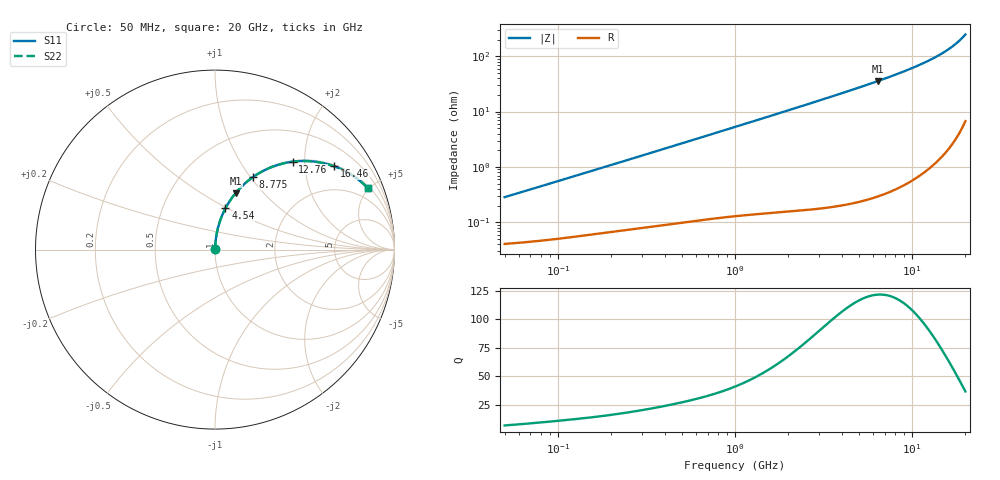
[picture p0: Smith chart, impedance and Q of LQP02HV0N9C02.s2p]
!Murata Part Number: LQP02HV0N9C02
!These Parameters are Measured in Series Mode Connection
!  o--[Z]--o
!Port1  Port2
!  o-------o
!Freq. Start=50[MHz] Stop=20[GHz], 401[Steps]
# Hz S RI R 50
!Freq.(Hz) S11(Real) S11(Imag) S21(Real) S21(Imag) S12(Real) S12(Imag) S22(Real) S22(Imag)
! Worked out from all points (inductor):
!   401 points, 50 MHz to 20 GHz, reference 50 ohm
!   read as one part in series: L = 889 pH near 51.52 MHz
!   highest Q = 121 at 6.407 GHz (marker M1), where L = 884 pH
!   S11 on the Smith chart (normalised r, x): 50 MHz: 1.00, +0.01; 4.54 GHz: 1.00, +0.49; 8.775 GHz: 1.01, +1.03; 12.76 GHz: 1.02, +1.74; 16.46 GHz: 1.05, +2.82; 20 GHz: 1.13, +4.94
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5e7  0.000415 0.00281  0.9996 -0.00281  0.9996 -0.00281  0.000415 0.00281
1.364002e8  0.000625 0.00746  0.9994 -0.00746  0.9994 -0.00746  0.000625 0.00746
3.721004e8  0.00126 0.0198  0.9987 -0.0198  0.9987 -0.0198  0.00126 0.0198
1e9  0.00405 0.0524  0.996 -0.0524  0.996 -0.0524  0.00405 0.0524
1.714689e9  0.00954 0.0892  0.9905 -0.0892  0.9905 -0.0892  0.00954 0.0892
2.728004e9  0.022 0.1408  0.978 -0.1408  0.978 -0.1408  0.022 0.1408
3.519108e9  0.0356 0.1803  0.9644 -0.1803  0.9644 -0.1803  0.0356 0.1803
4.539627e9  0.0582 0.2297  0.9418 -0.2297  0.9418 -0.2297  0.0582 0.2297
5.433528e9  0.0827 0.2713  0.9173 -0.2713  0.9173 -0.2713  0.0827 0.2713
6.406762e9  0.1143 0.3141  0.8857 -0.3141  0.8857 -0.3141  0.1143 0.3141
7.442007e9  0.1535 0.3564  0.8465 -0.3564  0.8465 -0.3564  0.1535 0.3564
8.774992e9  0.2121 0.4045  0.7879 -0.4045  0.7879 -0.4045  0.2121 0.4045
9.745021e9  0.26 0.4341  0.74 -0.4341  0.74 -0.4341  0.26 0.4341
1.066139e10  0.3091 0.4573  0.6909 -0.4573  0.6909 -0.4573  0.3091 0.4573
1.166392e10  0.3663 0.4766  0.6337 -0.4766  0.6337 -0.4766  0.3663 0.4766
1.276073e10  0.4323 0.4897  0.5677 -0.4897  0.5677 -0.4897  0.4323 0.4897
1.460232e10  0.5477 0.491  0.4523 -0.491  0.4523 -0.491  0.5477 0.491
1.550395e10  0.6044 0.4816  0.3956 -0.4816  0.3956 -0.4816  0.6044 0.4816
1.646126e10  0.6634 0.4644  0.3366 -0.4644  0.3366 -0.4644  0.6634 0.4644
1.800918e10  0.7534 0.4211  0.2466 -0.4211  0.2466 -0.4211  0.7534 0.4211
1.940974e10  0.8256 0.3674  0.1744 -0.3674  0.1744 -0.3674  0.8256 0.3674
2e10  0.8526 0.3411  0.1474 -0.3411  0.1474 -0.3411  0.8526 0.3411
